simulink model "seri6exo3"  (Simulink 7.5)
settings: Solver=ode45  StartTime=0.0  StopTime=10  RelTol=1e-3

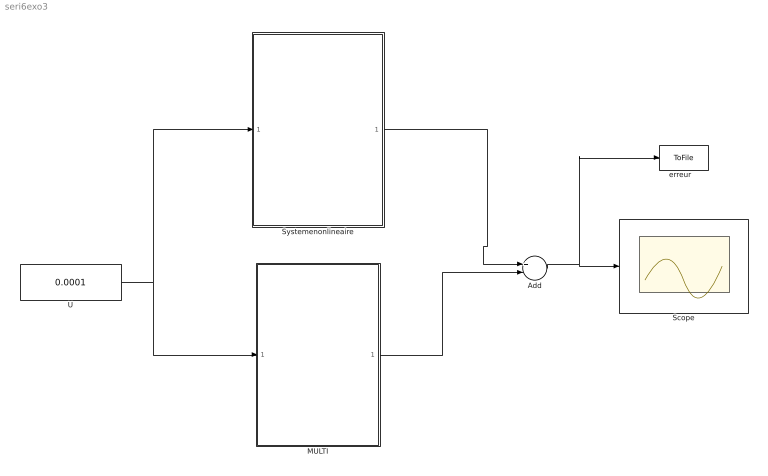
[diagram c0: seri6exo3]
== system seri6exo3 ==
  Add : Sum  Inputs=+-  OutDataType=fixdt(1, 16)  OutScaling=2^-10
  MULTI : Subsystem
  Scope : Scope
  Systemenonlineaire : Subsystem
  U : Constant  Value=0.0001  OutDataType=fixdt(1, 16)  OutScaling=2^0
  "erreur   " : ToFile  Filename=erreur
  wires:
  Systemenonlineaire/1(y) -> Add/1
  U/1 -> MULTI/1(U), Systemenonlineaire/1(u)
  Add/1 -> Scope/1, "erreur   "/1
  MULTI/1(Y) -> Add/2

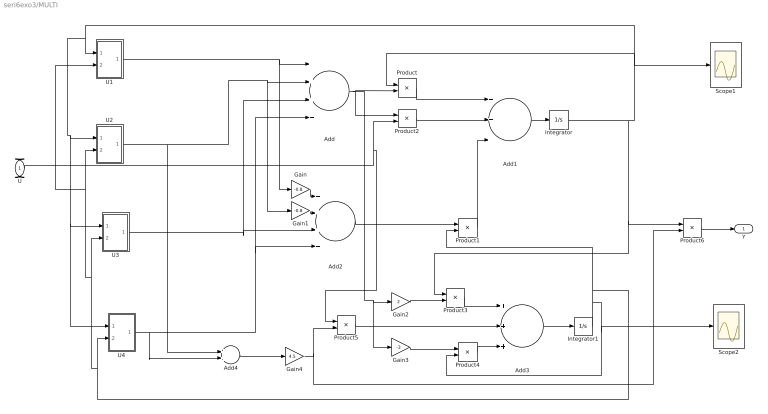
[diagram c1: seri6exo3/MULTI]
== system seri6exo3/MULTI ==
  U : Inport
  Add : Sum  Inputs=++++  OutDataType=fixdt(1, 16)  OutScaling=2^-10
  Add1 : Sum  Inputs=+++  OutDataType=fixdt(1, 16)  OutScaling=2^-10
  Add2 : Sum  Inputs=++++  OutDataType=fixdt(1, 16)  OutScaling=2^-10
  Add3 : Sum  Inputs=+++  OutDataType=fixdt(1, 16)  OutScaling=2^-10
  Add4 : Sum  OutDataType=fixdt(1, 16)  OutScaling=2^-10
  Gain : Gain  Gain=-0.8  ParameterDataType=fixdt(1, 16)  ParameterScaling=2^0  OutDataType=fixdt(1, 16)  OutScaling=2^0
  Gain1 : Gain  Gain=-0.8  ParameterDataType=fixdt(1, 16)  ParameterScaling=2^0  OutDataType=fixdt(1, 16)  OutScaling=2^0
  Gain2 : Gain  Gain=2  ParameterDataType=fixdt(1, 16)  ParameterScaling=2^0  OutDataType=fixdt(1, 16)  OutScaling=2^0
  Gain3 : Gain  Gain=-3  ParameterDataType=fixdt(1, 16)  ParameterScaling=2^0  OutDataType=fixdt(1, 16)  OutScaling=2^0
  Gain4 : Gain  Gain=4.5  ParameterDataType=fixdt(1, 16)  ParameterScaling=2^0  OutDataType=fixdt(1, 16)  OutScaling=2^0
  Integrator : Integrator
  Integrator1 : Integrator
  Product{,1..6} (7 alike) : Product  OutDataType=fixdt(1, 16)  OutScaling=2^0
  Scope1 : Scope
  Scope2 : Scope
  U1 : Subsystem
  U2 : Subsystem
  U3 : Subsystem
  U4 : Subsystem
  Y : Outport
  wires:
  U1/1(U1) -> Add/1, Gain/1
  U2/1(U2) -> Add/2, Gain1/1, Add4/1
  U3/1(U3) -> Add/3, Add2/3
  U4/1(U4) -> Add/4, Add2/4, Add4/2
  Add1/1 -> Integrator/1
  Integrator/1 -> Product/1, U1/1(X1), U2/1(In1), U3/1(X1), U4/1(X1), Scope1/1, Product3/1, Product6/1
  Add/1 -> Product/2, Product2/1, Gain2/1, Gain3/1
  Product/1 -> Add1/1
  Gain/1 -> Add2/1
  Gain1/1 -> Add2/2
  Add2/1 -> Product1/1
  Integrator1/1 -> Product1/2, U4/2(X2), U3/2(X2), U2/2(X2), U1/2(X2), Product4/2, Scope2/1
  Product1/1 -> Add1/3
  U/1 -> Product5/1, Product2/2
  Product2/1 -> Add1/2
  Gain2/1 -> Product3/2
  Product3/1 -> Add3/1
  Add3/1 -> Integrator1/1
  Gain3/1 -> Product4/1
  Product4/1 -> Add3/3
  Add4/1 -> Gain4/1
  Gain4/1 -> Product5/2, Product6/2
  Product5/1 -> Add3/2
  Product6/1 -> Y/1

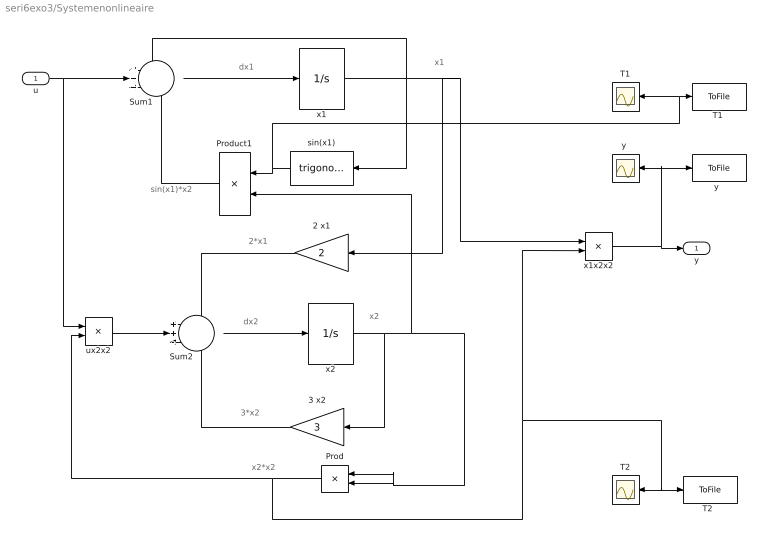
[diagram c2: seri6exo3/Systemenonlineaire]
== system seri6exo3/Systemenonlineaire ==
  note: dx1
  note: dx2
  note: x1
  note: x2
  note: x2*x2
  note: 3*x2
  note: 2*x1
  note: sin(x1)*x2
  u : Inport
  2 x1 : Gain  Gain=2  ParameterDataType=fixdt(1, 16)  ParameterScaling=2^0  OutDataType=fixdt(1, 16)  OutScaling=2^0
  3 x2 : Gain  Gain=3  ParameterDataType=fixdt(1, 16)  ParameterScaling=2^0  OutDataType=fixdt(1, 16)  OutScaling=2^0
  Prod : Product  OutDataType=fixdt(1, 16)  OutScaling=2^0
  Product1 : Product  OutDataType=fixdt(1, 16)  OutScaling=2^0
  Sum1 : Sum  Inputs=+++  OutDataType=fixdt(1, 16)  OutScaling=2^0
  Sum2 : Sum  Inputs=++-  OutDataType=fixdt(1, 16)  OutScaling=2^0
  T1 : Scope
  "T1 " : ToFile  Filename=terme1
  T2 : Scope
  "T2  " : ToFile  Filename=terme2
  sin(x1) : Trigonometry
  ux2x2 : Product  OutDataType=fixdt(1, 16)  OutScaling=2^0
  x1 : Integrator
  x1x2x2 : Product  OutDataType=fixdt(1, 16)  OutScaling=2^0
  x2 : Integrator
  "y " : Scope
  "y  " : ToFile  Filename=sortie
  y : Outport
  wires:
  Sum1/1 -> x1/1
  x1/1 -> sin(x1)/1, Sum1/1, 2 x1/1, x1x2x2/1
  sin(x1)/1 -> Product1/1, T1/1, "T1 "/1
  Sum2/1 -> x2/1
  x2/1 -> Product1/2, Prod/2, Prod/1, 3 x2/1
  Product1/1 -> Sum1/3
  u/1 -> ux2x2/1, Sum1/2
  2 x1/1 -> Sum2/1
  3 x2/1 -> Sum2/3
  Prod/1 -> ux2x2/2, x1x2x2/2, T2/1, "T2  "/1
  ux2x2/1 -> Sum2/2
  x1x2x2/1 -> y/1, "y "/1, "y  "/1

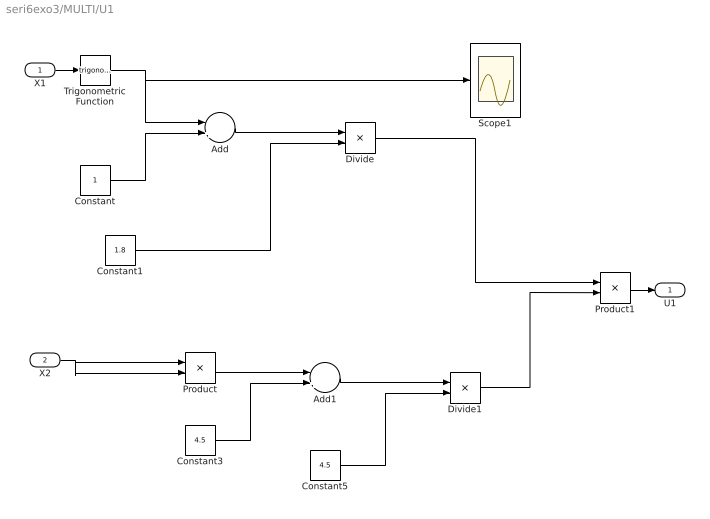
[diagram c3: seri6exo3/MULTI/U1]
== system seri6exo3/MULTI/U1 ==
  X1 : Inport
  X2 : Inport  Port=2
  Add : Sum  Inputs=-+  OutDataType=fixdt(1, 16)  OutScaling=2^-10
  Add1 : Sum  Inputs=-+  OutDataType=fixdt(1, 16)  OutScaling=2^-10
  Constant : Constant  OutDataType=fixdt(1, 16)  OutScaling=2^0
  Constant1 : Constant  Value=1.8  OutDataType=fixdt(1, 16)  OutScaling=2^0
  Constant3 : Constant  Value=4.5  OutDataType=fixdt(1, 16)  OutScaling=2^0
  Constant5 : Constant  Value=4.5  OutDataType=fixdt(1, 16)  OutScaling=2^0
  Divide : Product  Inputs=*/  OutDataType=fixdt(1, 16)  OutScaling=2^-10
  Divide1 : Product  Inputs=*/  OutDataType=fixdt(1, 16)  OutScaling=2^-10
  Product : Product  OutDataType=fixdt(1, 16)  OutScaling=2^0
  Product1 : Product  OutDataType=fixdt(1, 16)  OutScaling=2^0
  Scope1 : Scope
  Trigonometric Function : Trigonometry
  U1 : Outport
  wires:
  X2/1 -> Product/1, Product/2
  Product/1 -> Add1/1
  Constant3/1 -> Add1/2
  Add1/1 -> Divide1/1
  Constant5/1 -> Divide1/2
  Divide1/1 -> Product1/2
  Divide/1 -> Product1/1
  X1/1 -> Trigonometric Function/1
  Product1/1 -> U1/1
  Constant1/1 -> Divide/2
  Add/1 -> Divide/1
  Constant/1 -> Add/2
  Trigonometric Function/1 -> Add/1, Scope1/1

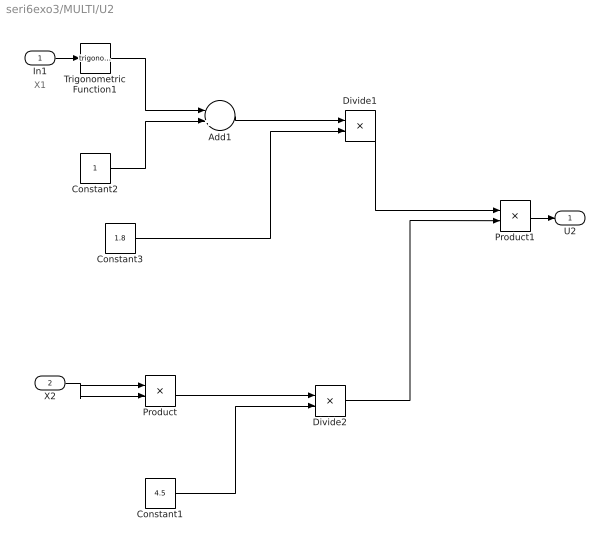
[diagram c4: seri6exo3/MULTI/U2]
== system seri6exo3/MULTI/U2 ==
  note: X1
  In1 : Inport
  X2 : Inport  Port=2
  Add1 : Sum  Inputs=-+  OutDataType=fixdt(1, 16)  OutScaling=2^-10
  Constant1 : Constant  Value=4.5  OutDataType=fixdt(1, 16)  OutScaling=2^0
  Constant2 : Constant  OutDataType=fixdt(1, 16)  OutScaling=2^0
  Constant3 : Constant  Value=1.8  OutDataType=fixdt(1, 16)  OutScaling=2^0
  Divide1 : Product  Inputs=*/  OutDataType=fixdt(1, 16)  OutScaling=2^-10
  Divide2 : Product  Inputs=*/  OutDataType=fixdt(1, 16)  OutScaling=2^-10
  Product : Product  OutDataType=fixdt(1, 16)  OutScaling=2^0
  Product1 : Product  OutDataType=fixdt(1, 16)  OutScaling=2^0
  Trigonometric Function1 : Trigonometry
  U2 : Outport
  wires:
  Constant3/1 -> Divide1/2
  Add1/1 -> Divide1/1
  Constant2/1 -> Add1/2
  Trigonometric Function1/1 -> Add1/1
  X2/1 -> Product/1, Product/2
  Product/1 -> Divide2/1
  Constant1/1 -> Divide2/2
  Divide1/1 -> Product1/1
  Divide2/1 -> Product1/2
  In1/1 -> Trigonometric Function1/1
  Product1/1 -> U2/1

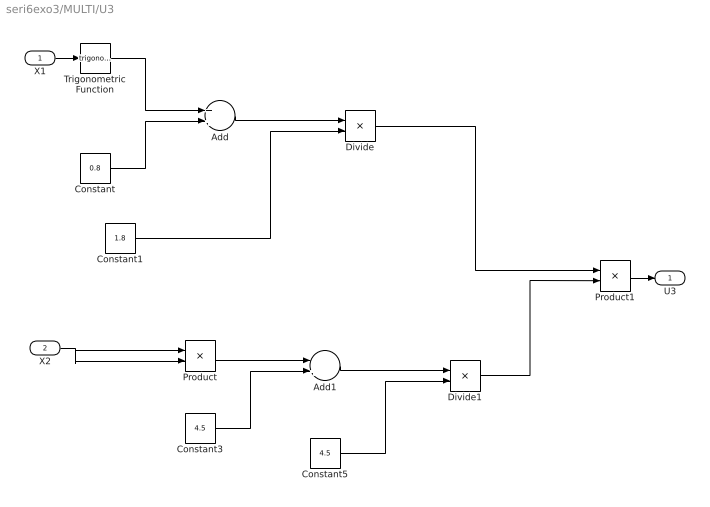
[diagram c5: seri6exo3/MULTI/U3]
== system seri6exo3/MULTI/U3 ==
  X1 : Inport
  X2 : Inport  Port=2
  Add : Sum  OutDataType=fixdt(1, 16)  OutScaling=2^-10
  Add1 : Sum  Inputs=-+  OutDataType=fixdt(1, 16)  OutScaling=2^-10
  Constant : Constant  Value=0.8  OutDataType=fixdt(1, 16)  OutScaling=2^0
  Constant1 : Constant  Value=1.8  OutDataType=fixdt(1, 16)  OutScaling=2^0
  Constant3 : Constant  Value=4.5  OutDataType=fixdt(1, 16)  OutScaling=2^0
  Constant5 : Constant  Value=4.5  OutDataType=fixdt(1, 16)  OutScaling=2^0
  Divide : Product  Inputs=*/  OutDataType=fixdt(1, 16)  OutScaling=2^-10
  Divide1 : Product  Inputs=*/  OutDataType=fixdt(1, 16)  OutScaling=2^-10
  Product : Product  OutDataType=fixdt(1, 16)  OutScaling=2^0
  Product1 : Product  OutDataType=fixdt(1, 16)  OutScaling=2^0
  Trigonometric Function : Trigonometry
  U3 : Outport
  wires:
  X2/1 -> Product/1, Product/2
  Product/1 -> Add1/1
  Constant3/1 -> Add1/2
  Add1/1 -> Divide1/1
  Constant5/1 -> Divide1/2
  Divide1/1 -> Product1/2
  Divide/1 -> Product1/1
  Constant1/1 -> Divide/2
  Add/1 -> Divide/1
  Constant/1 -> Add/2
  Trigonometric Function/1 -> Add/1
  X1/1 -> Trigonometric Function/1
  Product1/1 -> U3/1

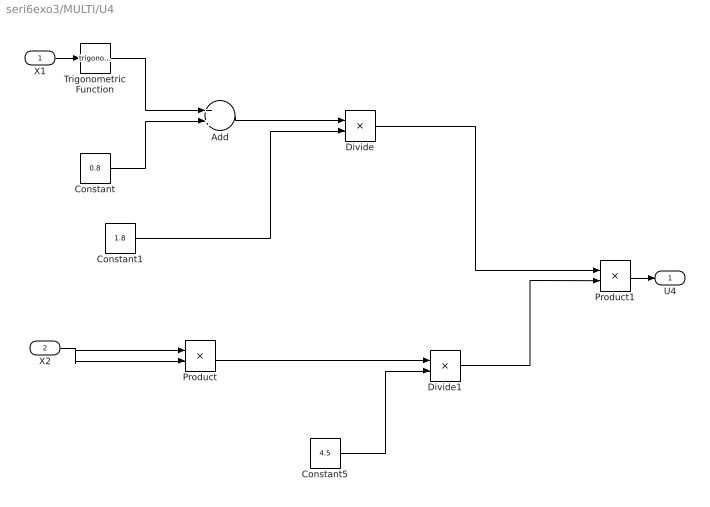
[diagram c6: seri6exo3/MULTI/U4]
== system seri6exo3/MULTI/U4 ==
  X1 : Inport
  X2 : Inport  Port=2
  Add : Sum  OutDataType=fixdt(1, 16)  OutScaling=2^-10
  Constant : Constant  Value=0.8  OutDataType=fixdt(1, 16)  OutScaling=2^0
  Constant1 : Constant  Value=1.8  OutDataType=fixdt(1, 16)  OutScaling=2^0
  Constant5 : Constant  Value=4.5  OutDataType=fixdt(1, 16)  OutScaling=2^0
  Divide : Product  Inputs=*/  OutDataType=fixdt(1, 16)  OutScaling=2^-10
  Divide1 : Product  Inputs=*/  OutDataType=fixdt(1, 16)  OutScaling=2^-10
  Product : Product  OutDataType=fixdt(1, 16)  OutScaling=2^0
  Product1 : Product  OutDataType=fixdt(1, 16)  OutScaling=2^0
  Trigonometric Function : Trigonometry
  U4 : Outport
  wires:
  Product1/1 -> U4/1
  X1/1 -> Trigonometric Function/1
  Trigonometric Function/1 -> Add/1
  Constant/1 -> Add/2
  Add/1 -> Divide/1
  Constant1/1 -> Divide/2
  Divide/1 -> Product1/1
  Divide1/1 -> Product1/2
  Constant5/1 -> Divide1/2
  X2/1 -> Product/2, Product/1
  Product/1 -> Divide1/1
